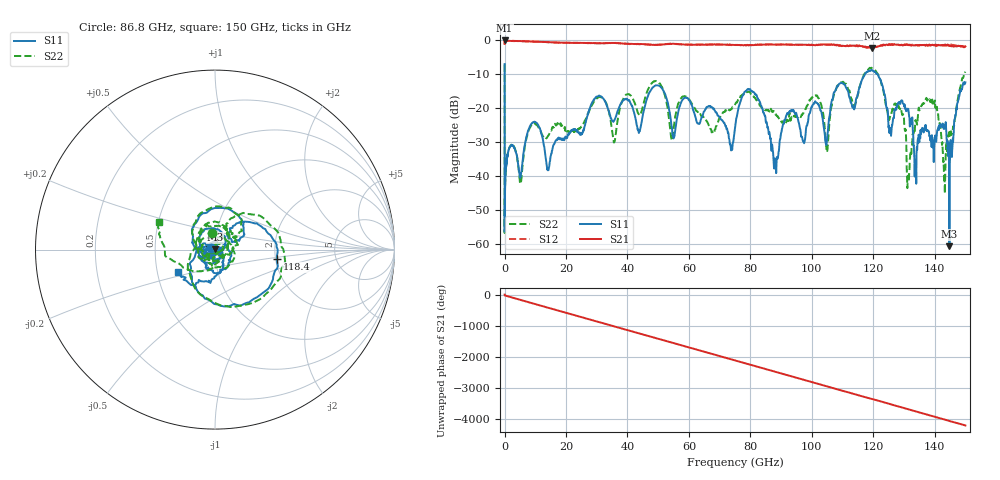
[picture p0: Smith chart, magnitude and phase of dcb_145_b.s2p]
! Filename: DCB145B.S2P
! Coder: SHF Communication Technologies
! IF Bandwidth: 10000 Hz
! Averaging: 0
! Smoothing: 0
! SourceAttenuator: 0 dB
! TestAttenuator: 0 dB
! SweepTime: 0 s
! ElectricalDelay: 0 s
# GHZ S DB R 50
! FREQ S11M S11A S21M S21A S12M S12A S22M S22A
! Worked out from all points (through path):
!   1913 points, 40 kHz to 150 GHz, reference 50 ohm
!   highest |S21| = 0.00 dB at 3.6 MHz (marker M1); lowest = -2.2 dB at 119.6 GHz (marker M2)
!   group delay of S21, straight-line fit = 77.8 ps
!   lowest |S11| = -60.6 dB at 144.8 GHz (marker M3), VSWR 1.00, Z = 50 + j0.0928 ohm
!   |S11| at or under -10 dB: 62.12 kHz to 117.3 GHz (117.3 GHz wide, 200 % of centre); 121.5 GHz to end of sweep
!   |S22| runs from -56.7 to -7.1 dB; largest |S21 - S12| = 0.087
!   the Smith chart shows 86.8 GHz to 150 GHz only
!   S11 on the Smith chart (normalised r, x): 86.8 GHz: 0.95, +0.02; 118.4 GHz: 2.04, -0.24; 150 GHz: 0.64, -0.17
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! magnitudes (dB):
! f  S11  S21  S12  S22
! 40 kHz  -7.0  -1.0  -1.0  -7.1
! 1 MHz  -33.4  0.0  0.0  -33.5
! 3.6 MHz  -45.1  0.0  0.0  -45.0
! 15 MHz  -56.3  0.0  0.0  -56.7
! 1 GHz  -33.5  -0.1  -0.1  -33.4
! 9.1 GHz  -24.3  -0.3  -0.3  -24.7
! 14.2 GHz  -38.2  -0.5  -0.5  -28.0
! 25.1 GHz  -27.2  -0.7  -0.7  -25.3
! 50.1 GHz  -13.3  -1.3  -1.2  -12.3
! 54.4 GHz  -25.3  -1.0  -1.0  -29.4
! 75.1 GHz  -25.2  -1.3  -1.3  -18.7
! 80.1 GHz  -14.8  -1.4  -1.3  -15.7
! 86.8 GHz  -31.7  -1.2  -1.2  -20.3
! 100.1 GHz  -19.5  -1.4  -1.3  -16.9
! 104.9 GHz  -29.7  -1.2  -1.2  -32.9
! 118.4 GHz  -9.1  -2.0  -2.1  -8.6
! 119.6 GHz  -8.7  -2.2  -2.0  -8.2
! 125.1 GHz  -25.2  -1.2  -1.2  -23.1
! 131.7 GHz  -22.4  -1.3  -1.3  -39.0
! 136.8 GHz  -25.6  -1.4  -1.3  -18.1
! 144.8 GHz  -60.6  -1.6  -1.3  -28.0
! 150 GHz  -12.3  -1.8  -1.6  -9.2
